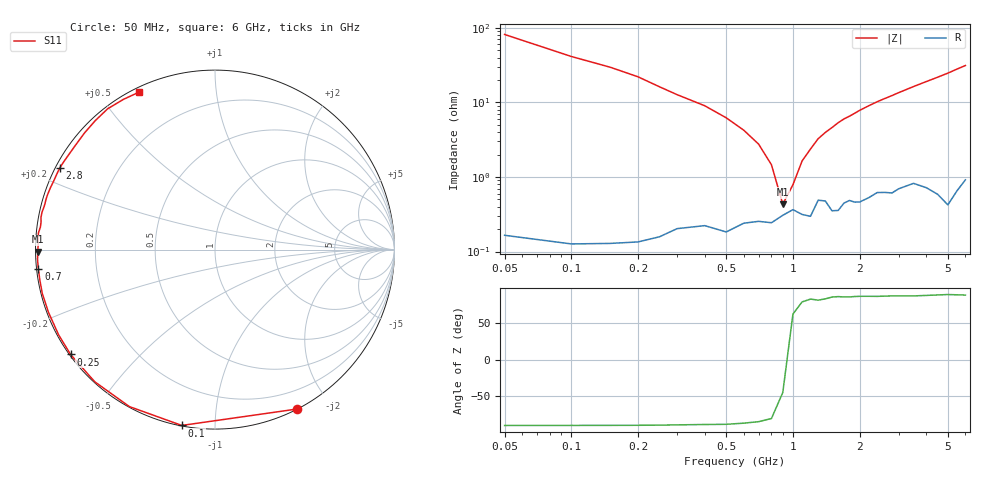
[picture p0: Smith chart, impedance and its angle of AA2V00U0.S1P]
! Infineon Technologies  Discrete & RF Semiconductors
! BBY66-02W
! Si Tuning Diode in SCD-80
! VR = 2 V
! S-Parameters:  June  2000
# GHz  S  MA  R  50
!  f  S11
! GHz  MAG  ANG
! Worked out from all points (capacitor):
!   34 points, 50 MHz to 6 GHz, reference 50 ohm
!   read as one part to ground: C = 38 pF near 50 MHz
!   lowest |Z| = 433 mohm at 900 MHz (marker M1)
!   series resonance near 930.4 MHz, so ESL is about 770 pH
!   S11 on the Smith chart (normalised r, x): 50 MHz: 0.00, -1.64; 100 MHz: 0.00, -0.83; 250 MHz: 0.00, -0.32; 700 MHz: 0.01, -0.06; 2.8 GHz: 0.01, +0.25; 6 GHz: 0.02, +0.63
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0.05  0.9982 -62.9
0.1  0.997 -100.7
0.15  0.9962 -118.6
0.2  0.9955 -132.3
0.25  0.9943 -144.0
0.3  0.9924 -151.4
0.4  0.9914 -159.5
0.5  0.9928 -165.8
0.6  0.9905 -170.3
0.7  0.9899 -173.7
0.8  0.9903 -176.7
0.9  0.9878 -179.3
1.1  0.9875 176.3
1.2  0.9882 174.6
1.3  0.9807 172.6
1.5  0.9861 169.5
1.6  0.986 167.8
1.7  0.9825 166.3
2  0.9821 162.2
2.4  0.9765 156.9
2.8  0.9772 152.2
3  0.9744 149.7
3.5  0.9707 143.8
4  0.9752 138.2
4.5  0.9805 132.8
5  0.9865 127.3
5.5  0.9803 121.4
6  0.974 115.9
